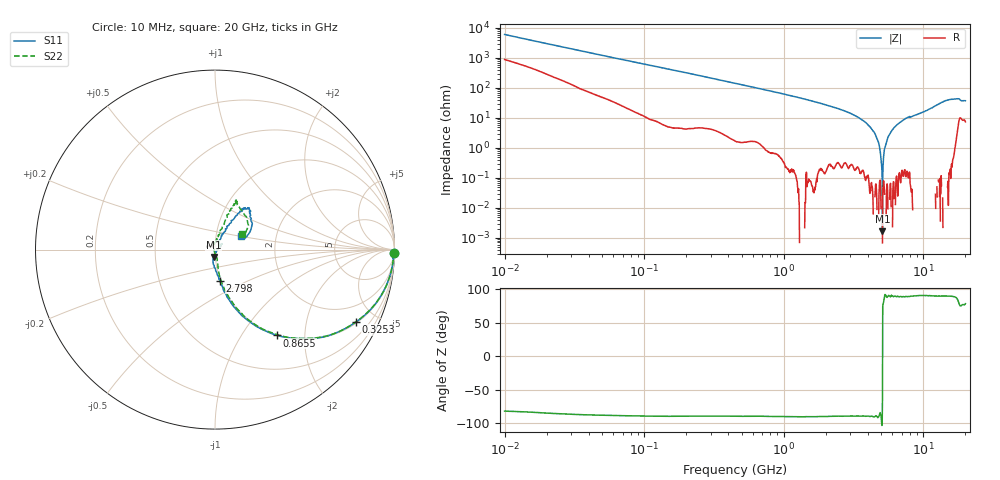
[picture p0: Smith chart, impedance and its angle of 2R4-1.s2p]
!Keysight Technologies,P5008B,MY61100088,A.16.20.02
!Date: Monday, May 27, 2024 14:33:25
!Correction: S11(C* 2-Port  )
!S21(C* 2-Port  )
!S12(C* 2-Port  )
!S22(C* 2-Port  )
!S2P File: Measurements: S11, S21, S12, S22:Log Frequency Sweep
# Hz S  dB  R 50
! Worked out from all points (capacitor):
!   1601 points, 10 MHz to 20 GHz, reference 50 ohm
!   read as one part in series: C = 2.67 pF near 10.39 MHz
!   lowest |Z| = 1.65 mohm at 5.091 GHz (marker M1)
!   series resonance near 5.092 GHz, so ESL is about 370 pH
!   S11 on the Smith chart (normalised r, x): 10 MHz: open; 325.3 MHz: 1.06, -3.89; 865.5 MHz: 0.99, -1.45; 2.798 GHz: 0.99, -0.35; 20 GHz: 1.32, +0.20
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1e7  -0.00 -0.9  -35.65 80.7  -35.67 80.7  -0.03 -0.9
3.555162e7  -0.04 -3.3  -24.62 83.6  -24.63 83.6  -0.05 -3.4
1.263918e8  -0.21 -11.4  -14.14 77.8  -14.16 77.8  -0.20 -11.4
3.253002e8  -1.07 -27.1  -6.89 61.9  -6.90 61.9  -1.08 -27.0
4.472136e8  -1.80 -35.2  -4.87 54.3  -4.88 54.3  -1.79 -35.0
8.655496e8  -4.59 -54.2  -1.90 35.6  -1.92 35.6  -4.59 -53.6
1.589917e9  -9.13 -70.7  -0.56 19.6  -0.57 19.6  -9.09 -69.6
2.798263e9  -15.13 -81.1  -0.13 8.2  -0.14 8.2  -15.09 -78.8
3.995989e9  -21.04 -93.1  -0.02 1.9  -0.03 2.0  -21.53 -79.0
5.091486e9  -27.55 -100.5  0.00 -2.3  -0.00 -2.3  -27.80 -81.3
5.652411e9  -33.78 -92.2  0.02 -4.1  0.01 -4.1  -33.52 -91.6
6.069891e9  -37.63 -44.4  0.03 -5.4  0.02 -5.4  -40.44 -112.3
6.335038e9  -38.08 -7.4  0.03 -6.2  0.02 -6.2  -45.35 -174.6
6.549245e9  -35.43 13.4  0.03 -6.8  0.02 -6.8  -39.61 147.1
7.066454e9  -30.30 28.1  0.03 -8.2  0.02 -8.2  -33.45 115.1
7.624508e9  -27.44 37.4  0.02 -9.7  0.02 -9.7  -28.99 106.8
8.344716e9  -28.97 37.7  0.04 -11.4  0.03 -11.4  -29.89 105.8
9.30816e9  -28.62 55.6  0.04 -13.8  0.03 -13.9  -28.24 92.9
1.400536e10  -12.03 56.5  -0.19 -26.0  -0.20 -26.1  -12.12 68.0
1.661757e10  -10.86 48.0  -0.36 -31.7  -0.37 -31.7  -10.89 64.0
1.871311e10  -15.38 21.8  -0.83 -33.0  -0.84 -33.0  -15.20 28.0
2e10  -15.87 27.5  -0.68 -33.8  -0.69 -33.8  -15.20 29.9
